(* Logix 5000 DataType export RTA_SCNDR_Dual_Scanner; software revision 32.00 *)

TYPE RTA_SCNDR_Dual_Scanner :
STRUCT
   Heartbeat : INT;   // Controller scope tag that the 435NBX updates with a free running counter to let the PLC know the 435NBX is present and actively communicating.
   Active : BOOL;   // Controller scope tag that the RTA_SCNDR_Heartbeat AOI uses to let the PLC show an active connection.
   P0_Received_Garbage_Data : BOOL;   // Controller scope tag that the RTA_SCNDR_P0_Barcode_Scanner_to_PLC AOI uses to indicate that it received data that was garbage. Potentially due to removal of cable to scanner or removal of power from the scanner.
   P1_Received_Garbage_Data : BOOL;   // Controller scope tag that the RTA_SCNDR_P1_Barcode_Scanner_to_PLC AOI uses to indicate that it received data that was garbage. Potentially due to removal of cable to scanner or removal of power from the scanner.
   P0_ASCII_Data : RTA_STRING_4096;   // Controller scope tag that the RTA 435NBX writes the ASCII data received from the barcode scanner on port 0 to the RTA_SCNDR_P0_Barcode_Scanner_to_PLC AOI
   P0_Barcode_Data : RTA_STRING_4096;   // Controller scope tag that the RTA_SCNDR_P0_Barcode_Scanner_to_PLC AOI uses to make data available to the PLC program.
   P1_ASCII_Data : RTA_STRING_4096;   // Controller scope tag that the RTA 435NBX writes the ASCII data received from the barcode scanner on port 1 to the RTA_SCNDR_P1_Barcode_Scanner_to_PLC AOI
   P1_Barcode_Data : RTA_STRING_4096;   // Controller scope tag that the RTA_SCNDR_P1_Barcode_Scanner_to_PLC AOI uses to make data available to the PLC program.
END_STRUCT
END_TYPE

TYPE RTA_STRING_4096 :   // string type; String data type with up to 4096 characters available.
STRUCT
   LEN : DINT;
   DATA : SINT[4096];
END_STRUCT
END_TYPE
